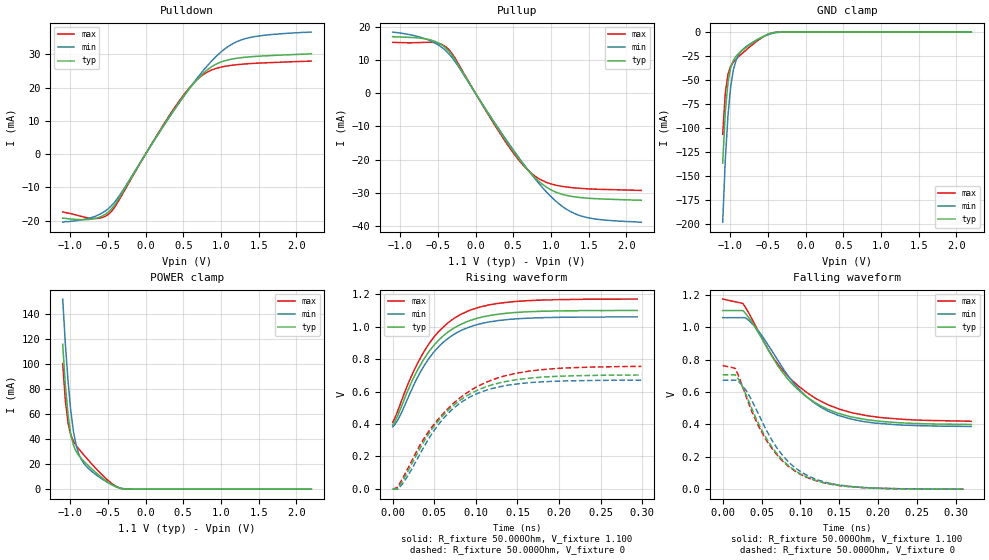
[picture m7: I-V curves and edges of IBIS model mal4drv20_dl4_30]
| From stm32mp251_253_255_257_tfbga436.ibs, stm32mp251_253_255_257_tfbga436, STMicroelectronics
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[Model] mal4drv20_dl4_30
Model_type   I/O
Polarity   Non-Inverting
Enable   Active-High
C_comp   1.837pF   1.837pF   1.849pF
C_comp_pullup   942.491fF   934.703fF   950.576fF
C_comp_pulldown 782.742fF   781.933fF   799.826fF
Vinh = 404.000mV
Vinl = 284.000mV
Vmeas = 344.000mV
Vref = 0.00V
Rref = 50Ohms
Cref = 0pF
[Model Spec]
Vinh   404.000mV   391.000mV   426.000mV
Vinl   284.000mV   271.000mV   306.000mV
Vmeas   344.000mV   331.000mV   366.000mV
Vref   0.00V   0.00V   0.00V
D_overshoot_ampl_h 0.3 NA   NA
D_overshoot_ampl_l 0.3 NA   NA
D_overshoot_area_l 100.000m NA   NA
D_overshoot_area_h 100.000m NA   NA
[Receiver Thresholds]
Vth = 344.000mV
Vth_min = 331.000mV
Vth_max = 366.000mV
Vinh_ac = 600.000mV
Vinh_dc = 600.000mV
Vinl_ac = -600.000mV
Vinl_dc = -600.000mV
Tslew_ac = 5.000ns
Threshold_sensitivity = 0.5
Reference_supply Pullup_ref
[Temperature Range]   25.000   125.000   -40.000
[Voltage Range]   1.100V   1.060V   1.170V
[GND Clamp Reference]   0.00V   0.00V   0.00V
[C Comp Corner]
| variable   typ   min   max
C_comp 1.849pF   1.837pF   1.837pF
C_comp_pullup 942.491fF   950.576fF   934.703fF
C_comp_pulldown 781.933fF   799.826fF   782.742fF
[Pulldown Reference]   0.00V   0.00V   0.00V
[POWER Clamp Reference]   1.100V   1.060V   1.170V
[Pullup Reference]   1.100V   1.060V   1.170V
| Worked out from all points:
|   slope of the pulldown table from 0 to 0.165 V, typ, clamps not added: 27.5 ohm
|   slope of the pullup table from 0 to 0.165 V, typ, clamps not added: 27.5 ohm
|   GND clamp passes 1 mA (typ) near -0.45 V on its own axis
|   POWER clamp passes 1 mA (typ) near -0.36 V on its own axis
|   rising waveform, R_fixture 50.000Ohm, V_fixture 1.100: 20-80 % time 51.9ps typ, 51ps min, 53.3ps max; typ from 0.392 V to 1.1 V
|   rising waveform, R_fixture 50.000Ohm, V_fixture 0: 20-80 % time 63.8ps typ, 58.9ps min, 72.1ps max; typ from -0.001 V to 0.702 V
|   falling waveform, R_fixture 50.000Ohm, V_fixture 1.100: 20-80 % time 70.5ps typ, 67.4ps min, 75.7ps max; typ from 1.1 V to 0.4 V
|   falling waveform, R_fixture 50.000Ohm, V_fixture 0: 20-80 % time 54ps typ, 54.2ps min, 54.5ps max; typ from 0.707 V to 0 V
[GND Clamp]
-1.099V   -136.3mA   -197.9mA   -106.5mA
-1.064V   -82.47mA   -132mA     -62.93mA
-1.028V   -52.05mA   -85.75mA   -43.61mA
-992.7mV  -36.88mA   -56.43mA   -35.5mA
-957.3mV  -29.36mA   -39.14mA   -31.26mA
-921.8mV  -25.1mA    -29.22mA   -28.2mA
-886.4mV  -22.16mA   -23.33mA   -25.51mA
-850.9mV  -19.73mA   -19.54mA   -22.95mA
-780mV    -15.43mA   -14.59mA   -18.04mA
-531.8mV  -3.288mA   -3.748mA   -3.604mA
-390mV    -251.1uA   -613.4uA   -163.8uA
2.198V    42.3nA     621.2nA    4.643nA
[Power Clamp]
-1.098V   115.5mA    151.6mA    100.1mA
-1.063V   83.06mA    116mA      70.82mA
-1.027V   59.24mA    86.19mA    52.7mA
-991.8mV  44.02mA    63.02mA    43.29mA
-956.4mV  35.26mA    46.38mA    38.3mA
-920.9mV  30.19mA    35.27mA    34.98mA
-885.5mV  26.87mA    28.15mA    32.19mA
-850mV    24.29mA    23.52mA    29.6mA
-672.7mV  13.97mA    12.28mA    17.45mA
-424.5mV  2.786mA    2.91mA     3.554mA
-282.7mV  160.9uA    380.1uA    143.1uA
2.199V    -14.13nA   -533.6nA   -2.884nA
[Pulldown]
-1.099V   -19.3mA    -20.5mA    -17.4mA
-673.6mV  -19.41mA   -18.76mA   -19.39mA
-567.3mV  -18.57mA   -17.61mA   -19.05mA
-460.9mV  -16.73mA   -15.73mA   -17.46mA
-319.1mV  -12.05mA   -11.56mA   -12.55mA
106.4mV   3.9mA      3.8mA      4.043mA
425.4mV   14.91mA    14.76mA    15.29mA
673.6mV   22.16mA    22.53mA    22.21mA
850.9mV   25.9mA     27.37mA    25.04mA
1.099V    28.36mA    32.42mA    26.57mA
1.312V    29.12mA    34.65mA    27.1mA
2.198V    30.2mA     36.7mA     27.97mA
[Pullup]
-1.098V   17.1mA     18.49mA    15.4mA
-601.8mV  16.14mA    15.9mA     15.42mA
-460mV    14.8mA     14.09mA    14.86mA
-353.6mV  12.73mA    11.94mA    13.22mA
-247.3mV  9.26mA     8.791mA    9.708mA
461.8mV   -16.19mA   -15.8mA    -16.73mA
674.5mV   -22.6mA    -22.46mA   -22.74mA
851.8mV   -26.8mA    -27.5mA    -25.92mA
1.1V      -30.12mA   -33.22mA   -27.89mA
1.348V    -31.35mA   -36.61mA   -28.61mA
1.632V    -31.83mA   -38.06mA   -28.96mA
2.199V    -32.3mA    -38.9mA    -29.31mA
[Ramp]
R_load=50.000Ohm
dV/dt_r   421.350mV/59.000ps  403.229mV/55.500ps  452.610mV/64.000ps
dV/dt_f   421.350mV/63.500ps  403.229mV/62.000ps  452.610mV/66.500ps
[Rising waveform]
R_fixture=50.000Ohm
V_fixture=1.100
V_fixture_min=1.060
V_fixture_max=1.170
0s        392.3mV    383.6mV    410.4mV
6ps       451.3mV    423.7mV    480.1mV
10ps      501.7mV    463.2mV    535.5mV
23ps      662.2mV    614.8mV    700.8mV
39ps      812.2mV    769.2mV    857.9mV
58ps      930.3mV    890.6mV    983.7mV
82ps      1.014V     975.6mV    1.076V
108ps     1.06V      1.021V     1.125V
149ps     1.088V     1.048V     1.156V
294ps     1.1V       1.06V      1.17V
[Rising waveform]
R_fixture=50.000Ohm
V_fixture=0
0s        -885.3uV   -1.371mV   -290.5uV
5ps       -885.3uV   -1.371mV   7.054mV
15ps      76.76mV    54.97mV    94.06mV
37ps      287.5mV    254mV      306.1mV
59ps      443.9mV    422.8mV    454.8mV
80ps      543.1mV    525.1mV    557.4mV
108ps     621.7mV    600.6mV    647.4mV
136ps     662mV      637mV      698.4mV
183ps     690.1mV    661.1mV    737mV
299ps     702.2mV    670.2mV    755.1mV
[Falling waveform]
R_fixture=50.000Ohm
V_fixture=1.100
V_fixture_min=1.060
V_fixture_max=1.170
0s        1.104V     1.06V      1.175V
26ps      1.104V     1.06V      1.148V
35ps      1.052V     1.037V     1.076V
59ps      857.3mV    887.3mV    859.4mV
81ps      697.1mV    722.5mV    713.8mV
107ps     574.2mV    575.5mV    601.3mV
134ps     496mV      486.5mV    525.1mV
162ps     451mV      436.8mV    478.3mV
195ps     423.7mV    409.1mV    448.3mV
320ps     400.1mV    388mV      419.9mV
[Falling waveform]
R_fixture=50.000Ohm
V_fixture=0
0s        707.1mV    673.3mV    764.4mV
16ps      707.1mV    673.3mV    747.2mV
26ps      626.9mV    637.7mV    628mV
40ps      469.2mV    524.1mV    452.2mV
59ps      292.2mV    339.9mV    281.5mV
81ps      161mV      187mV      156.3mV
105ps     82.96mV    94.79mV    79.59mV
132ps     38.46mV    43.24mV    37.22mV
163ps     16.03mV    17.65mV    15.82mV
310ps     305.8uV    343.5uV    314.6uV
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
